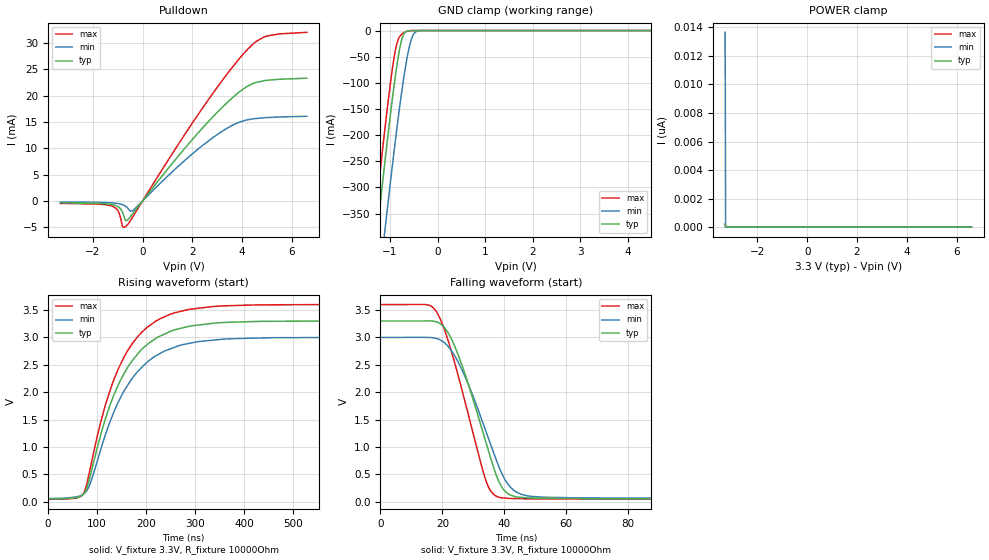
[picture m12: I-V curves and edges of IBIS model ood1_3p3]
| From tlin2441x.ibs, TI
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|   ood1_3p3 Model
[Model]   ood1_3p3
Model_type   Open_drain
Polarity   Non-Inverting
Vmeas = 1.65
Vref = 3.3
Cref = 2pF
Rref = 10000
|   typ   min   max
C_comp   4.760pF   4.567pF   4.782pF
|  Where Nom  PVT is Nominal Process, 3.3V,   27C
|   Fast PVT is Strong Process,  3.6,   -40C
|   Slow PVT is Weak Process,   3.0V,   150C
[Voltage Range]   3.3   3   3.6
|Junction Temperature
[Temperature Range]   27   150   -40
[Pullup Reference]   3.3   3   3.6
[Pulldown Reference]   0   0   0
[Power Clamp Reference]   3.3   3   3.6
[GND Clamp Reference]   0   0   0
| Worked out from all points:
|   slope of the pulldown table from 0 to 0.495 V, typ, clamps not added: 164 ohm
|   GND clamp passes 1 mA (typ) near -0.63 V on its own axis
|   falling waveform, V_fixture 3.3V, R_fixture 10000Ohm: 20-80 % time 10.8ns typ, 11.9ns min, 10ns max; typ from 3.3 V to 0.053 V
|   rising waveform, V_fixture 3.3V, R_fixture 10000Ohm: 20-80 % time 86.2ns typ, 89.4ns min, 82.6ns max; typ from 0.053 V to 3.3 V
[Pulldown]
|   Voltage   I(typ)   I(min)   I(max)
-3.3V     -352.8uA   -232.8uA   -465.8uA
-1.221V   -699.4uA   -370.9uA   -986.1uA
-993.3mV  -1.064mA   -484uA     -1.824mA
-894.3mV  -1.453mA   -573uA     -3.003mA
-815.1mV  -2.036mA   -681.6uA   -4.722mA
-676.5mV  -3.722mA   -1.023mA   -4.837mA
-399.3mV  -2.447mA   -1.872mA   -3.056mA
2.353V    13.57mA    10.33mA    17.26mA
3.382V    18.62mA    13.78mA    24.04mA
4.155V    21.63mA    15.36mA    28.49mA
4.966V    22.92mA    15.84mA    31.31mA
6.6V      23.34mA    16.1mA     32.06mA
[GND Clamp]
|   Voltage   I(typ)   I(min)   I(max)
-3.3V     -2.208A    -2.295A    -2.167A
-1.33V    -437.1mA   -567.1mA   -373.9mA
-1.231V   -353.3mA   -484.2mA   -289.5mA
-1.102V   -247.4mA   -378.6mA   -184.1mA
-983.4mV  -155mA     -284.1mA   -95.43mA
-884.4mV  -85.49mA   -208.8mA   -36.49mA
-815.1mV  -44.44mA   -158.9mA   -14.4mA
-765.6mV  -21.85mA   -125.3mA   -8.203mA
-666.6mV  -2.365mA   -65.63mA   -2.117mA
-537.9mV  -95.72uA   -13.62mA   -108.3uA
-399.3mV  -1.856uA   -548.8uA   -1.062uA
6.6V      0A         0A         0A
[POWER Clamp]
|   Voltage   I(typ)   I(min)   I(max)
-3.3V     204.9pA    13.66nA    207.2pA
-3.28V    0A         0A         0A
-3.27V    0A         0A         0A
6.6V      0A         0A         0A
[Ramp]
R_load = 10000
|   typ   min   max
dV/dt_r   1.94827/8.57183e-08   1.76342/8.92071e-08   2.13221/8.2679e-08
dV/dt_f   1.94827/1.08042e-08   1.76342/1.18798e-08   2.13221/1.00404e-08
[Falling Waveform]
V_fixture = 3.3V
V_fixture_min = 3V
V_fixture_max = 3.6V
R_fixture = 10000Ohm
C_fixture = 0F
|   Time   V(typ)   V(min)   V(max)
0s        3.3V       3V         3.6V
15.73ns   3.301V     2.999V     3.589V
18.21ns   3.284V     2.98V      3.457V
20.71ns   3.178V     2.9V       3.134V
26.5ns    2.466V     2.388V     2.003V
35.03ns   904.3mV    1.134V     253.6mV
37.76ns   434.5mV    712.6mV    95.29mV
40.24ns   194.6mV    403.6mV    68.44mV
47.91ns   72.13mV    105.9mV    55.33mV
5us       52.88mV    60.86mV    46.31mV
[Rising Waveform]
V_fixture = 3.3V
V_fixture_min = 3V
V_fixture_max = 3.6V
R_fixture = 10000Ohm
C_fixture = 0F
|   Time   V(typ)   V(min)   V(max)
0s        52.88mV    60.86mV    46.31mV
72.57ns   147.8mV    144.3mV    158.2mV
85.82ns   470.5mV    331.2mV    609.3mV
107.1ns   1.216V     949.4mV    1.448V
129.5ns   1.841V     1.535V     2.118V
155.4ns   2.346V     2.029V     2.65V
184.3ns   2.713V     2.393V     3.029V
247.8ns   3.103V     2.785V     3.417V
337.8ns   3.258V     2.951V     3.564V
5us       3.3V       3V         3.6V
